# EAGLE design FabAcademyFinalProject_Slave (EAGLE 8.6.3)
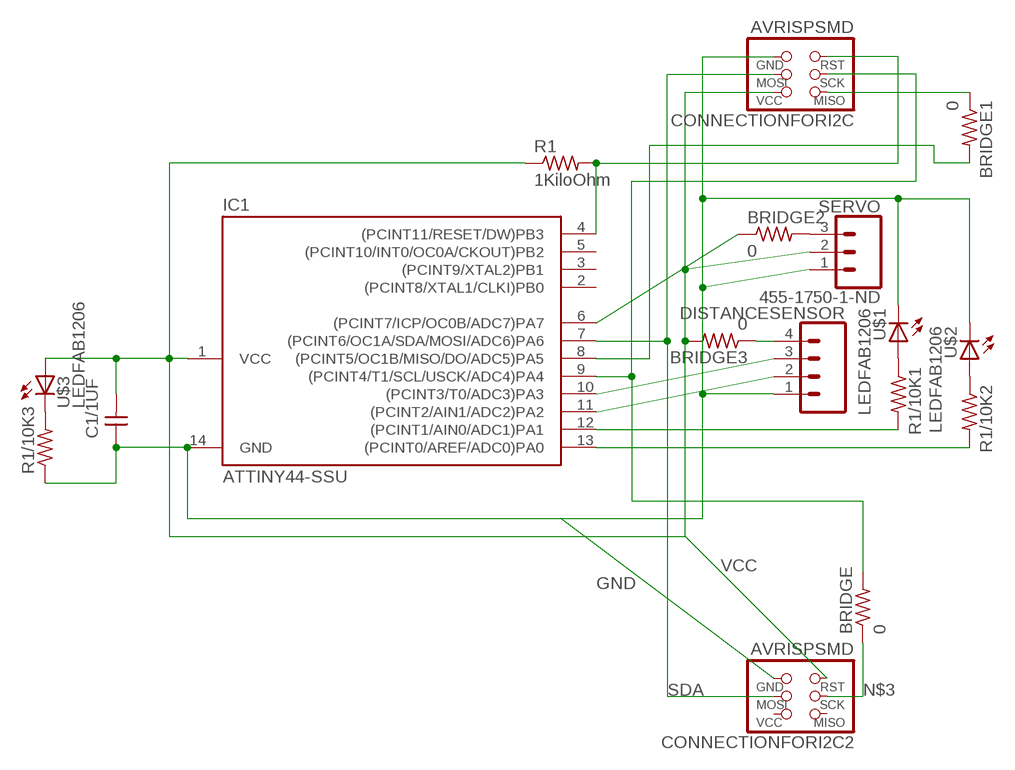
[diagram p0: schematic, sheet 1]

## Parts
BRIDGE  0  RES-US1206FAB  [R1206FAB]
BRIDGE1  0  RES-US1206FAB  [R1206FAB]
BRIDGE2  0  RES-US1206FAB  [R1206FAB]
BRIDGE3  0  RES-US1206FAB  [R1206FAB]
C1/1UF  CAP-UNPOLARIZEDFAB  [C1206FAB]
CONNECTIONFORI2C  AVRISPSMD  [2X03SMD]
CONNECTIONFORI2C2  AVRISPSMD  [2X03SMD]
DISTANCESENSOR  CONN_04  [1X04]
IC1  ATTINY44-SSU  [SOIC14]
R1  1KiloOhm  RES-US1206FAB  [R1206FAB]
R1/10K1  RES-US1206FAB  [R1206FAB]
R1/10K2  RES-US1206FAB  [R1206FAB]
R1/10K3  RES-US1206FAB  [R1206FAB]
SERVO  455-1750-1-ND  CONN_03  [1X03]
U$1  LEDFAB1206  [LED1206FAB]
U$2  LEDFAB1206  [LED1206FAB]
U$3  LEDFAB1206  [LED1206FAB]

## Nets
GND: C1/1UF.1 CONNECTIONFORI2C2.6(GND) CONNECTIONFORI2C.6(GND) DISTANCESENSOR.1 IC1.14(GND) R1/10K3.1 SERVO.1 U$1.2(C) U$2.2(C)
N$1: R1/10K2.1 U$2.1(A)
N$2: R1/10K3.2 U$3.2(C)
N$3: BRIDGE.1 CONNECTIONFORI2C2.3(SCK)
N$4: DISTANCESENSOR.3 IC1.10((PCINT3/T0/ADC3)PA3)
N$5: BRIDGE2.1 IC1.6((PCINT7/ICP/OC0B/ADC7)PA7)
N$6: BRIDGE1.2 IC1.8((PCINT5/OC1B/MISO/DO/ADC5)PA5)
N$7: CONNECTIONFORI2C.5(RST) IC1.4((PCINT11/RESET/DW)PB3) R1.2
N$8: IC1.13((PCINT0/AREF/ADC0)PA0) R1/10K2.2
N$9: IC1.12((PCINT1/AIN0/ADC1)PA1) R1/10K1.2
N$10: DISTANCESENSOR.2 IC1.11((PCINT2/AIN1/ADC2)PA2)
N$11: BRIDGE2.2 SERVO.3
N$12: R1/10K1.1 U$1.1(A)
N$13: BRIDGE3.1 DISTANCESENSOR.4
N$14: BRIDGE1.1 CONNECTIONFORI2C.1(MISO)
SCL: BRIDGE.2 CONNECTIONFORI2C.3(SCK) IC1.9((PCINT4/T1/SCL/USCK/ADC4)PA4)
SDA: CONNECTIONFORI2C2.4(MOSI) CONNECTIONFORI2C.4(MOSI) IC1.7((PCINT6/OC1A/SDA/MOSI/ADC6)PA6)
VCC: BRIDGE3.2 C1/1UF.2 CONNECTIONFORI2C2.5(RST) CONNECTIONFORI2C.2(VCC) IC1.1(VCC) R1.1 SERVO.2 U$3.1(A)
Unconnected: CONNECTIONFORI2C2.1(MISO) CONNECTIONFORI2C2.2(VCC) IC1.2((PCINT8/XTAL1/CLKI)PB0) IC1.3((PCINT9/XTAL2)PB1) IC1.5((PCINT10/INT0/OC0A/CKOUT)PB2)

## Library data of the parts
BRIDGE BRIDGE1-BRIDGE3 R1 R1/10K1-R1/10K3 = fab:RES-US: Resistor (US Symbol)
C1/1UF = fab:CAP-UNPOLARIZED
CONNECTIONFORI2C CONNECTIONFORI2C2 = fab:AVRISP
DISTANCESENSOR = SparkFun-Connectors:CONN_04: Multi connection point. Often used as Generic Header-pin footprint for 0.1 inch spaced/style header connections On any of the 0.1 inch spaced packages, you can populate with these: Break Away Headers - Straight (PRT-00116) Break Away Male Headers - Right Angle (PRT-00553) Female Headers (PRT-00115)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; PROD_ID: CONN-09696
IC1 = fab:ATTINY44
SERVO = SparkFun-Connectors:CONN_03: Multi connection point. Often used as Generic Header-pin footprint for 0.1 inch spaced/style header connections On any of the 0.1 inch spaced packages, you can populate with these: Break Away Headers - Straight (PRT-00116) Break Away Male Headers - Right Angle (PRT-00553) Female Headers (PRT-00115)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; PROD_ID: XXX-00000
U$1-U$3 = fab:LED: LED

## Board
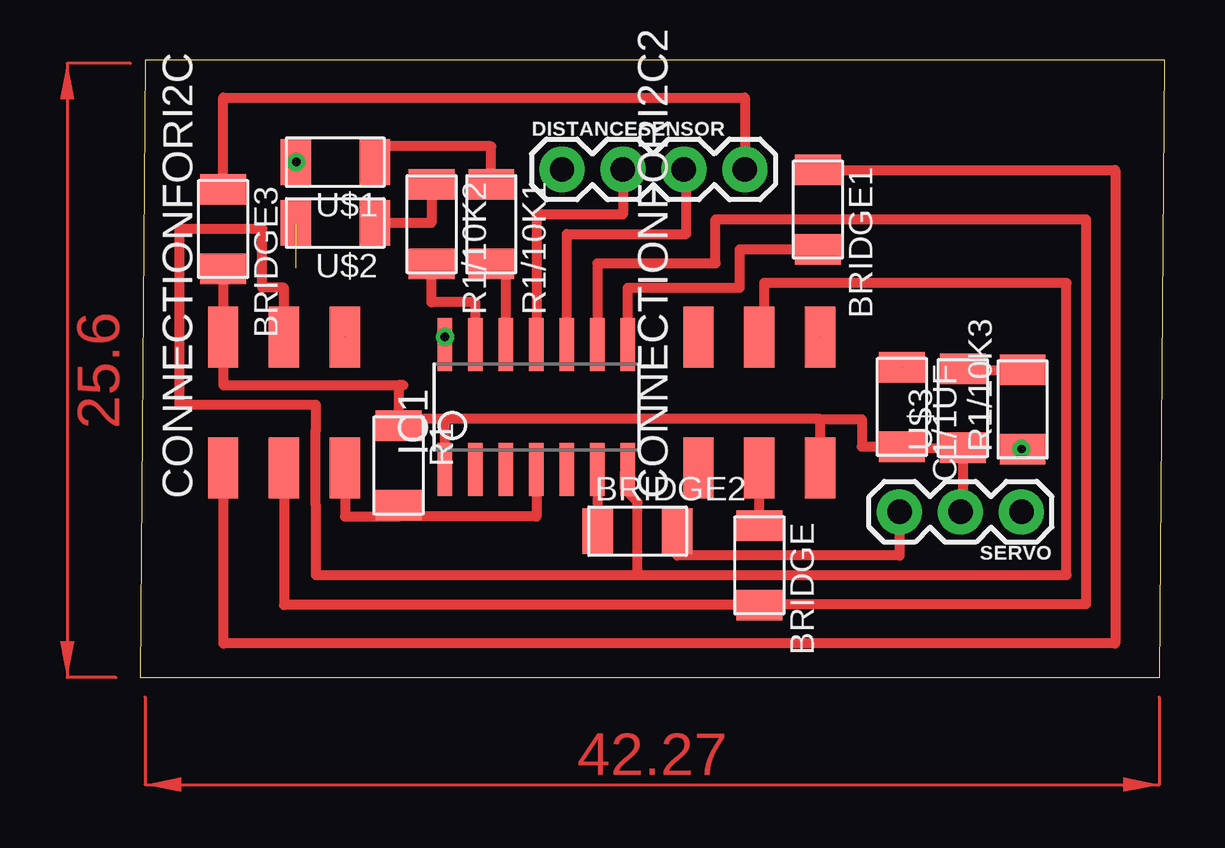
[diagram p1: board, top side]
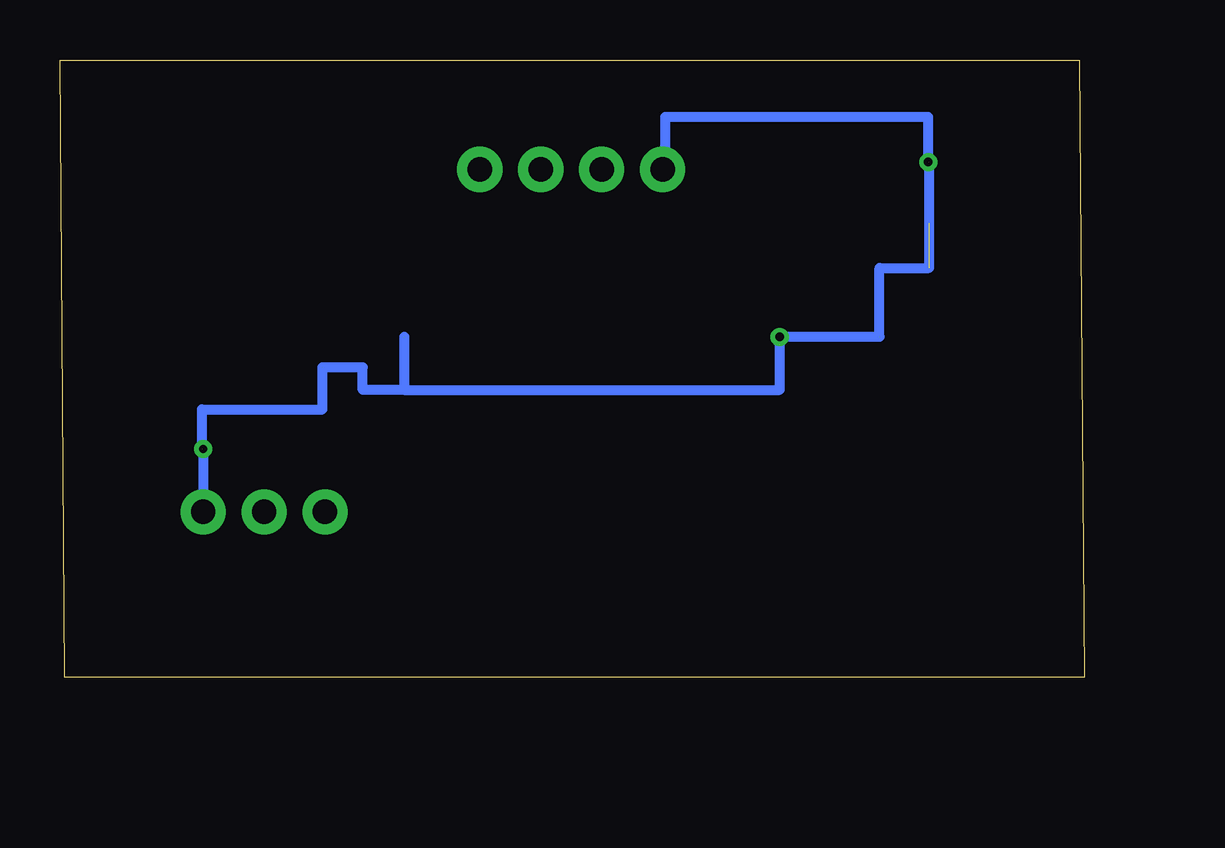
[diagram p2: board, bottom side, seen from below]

Size 42.7 x 25.75 mm. Coordinates in mm from the lower left corner, seen from the top.
Outline: 0,0 42.49,0 42.7,25.75 0.2,25.75 0,0
Copper layers (1*16): Top 0.035mm / dielectric 1.5mm / Bottom 0.035mm
Design rules "default *": minimum track width 6mil, minimum drill 0.35mm, track to track 16mil, track to pad 16mil, pad to pad 16mil, via to via 16mil, smd to smd 16mil, copper to edge 40mil, drill to drill 6mil, minimum pad ring 10mil, minimum via ring 8mil, stop-mask expansion 4mil, vias tented up to drill 0mil, thermal gap 10mil

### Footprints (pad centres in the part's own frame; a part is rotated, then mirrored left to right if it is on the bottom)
R1206FAB = smd 1.27 x 1.905: 1 -1.651,0; 2 1.651,0
C1206FAB = smd 1.27 x 1.905: 1 -1.651,0; 2 1.651,0
2X03SMD = smd 2.54 x 1.27: 1 -2.54,2.54; 2 2.92,2.54; 3 -2.54,0; 4 2.92,0; 5 -2.54,-2.54; 6 2.92,-2.54
1X04 = drill 1.016 pad 1.88: 1 0,0; 2 2.54,0; 3 5.08,0; 4 7.62,0
SOIC14 = smd 0.61 x 2.21: 1 -3.81,-2.603; 2 -2.54,-2.603; 3 -1.27,-2.603; 4 0,-2.603; 5 1.27,-2.603; 6 2.54,-2.603; 7 3.81,-2.603; 8 3.81,2.603; 9 2.54,2.603; 10 1.27,2.603; 11 0,2.603; 12 -1.27,2.603; 13 -2.54,2.603; 14 -3.81,2.603
1X03 = drill 1.016 pad 1.88: 1 0,0; 2 2.54,0; 3 5.08,0
LED1206FAB = smd 1.27 x 1.905: 1 -1.651,0; 2 1.651,0

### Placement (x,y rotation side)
BRIDGE  25.81,4.67 270 top
BRIDGE1  28.24,19.51 270 top
BRIDGE2  20.73,6.1 0 top
BRIDGE3  3.45,18.69 270 top
C1/1UF  31.75,11.28 270 top
CONNECTIONFORI2C  5.99,11.28 90 top
CONNECTIONFORI2C2  25.81,11.28 90 top
DISTANCESENSOR  17.58,21.18 0 top
IC1  16.51,11.28 0 top
R1  10.77,8.84 270 top
R1/10K1  14.63,18.9 270 top
R1/10K2  12.14,18.9 270 top
R1/10K3  36.78,11.18 90 top
SERVO  36.73,6.91 180 top
U$1  8.13,21.49 180 top
U$2  8.13,18.95 180 top
U$3  34.29,11.23 90 top

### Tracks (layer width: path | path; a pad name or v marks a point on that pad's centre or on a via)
GND  (via drill 0.35)  (7 unrouted)
  Top 0.406: v12.7,14.2 IC1.14 | R1/10K3.1 v36.73,9.52 | U$1.2 v6.5,21.49 | v17.48,21.18 DISTANCESENSOR.1
  Bottom 0.406: CONNECTIONFORI2C2.6 28.35,11.99 | 28.35,11.99 12.7,11.99 IC1.14 | 28.35,11.99 30.07,11.99 30.07,12.93 C1/1UF.1 31.75,11.18 36.78,11.18 R1/10K3.1 | U$1.2 6.48,17.07 8.53,17.07 CONNECTIONFORI2C.6 v12.7,14.2 | v36.73,9.52 SERVO.1 | v6.5,21.49 6.5,23.37 17.48,23.37 v17.48,21.18
N$1
  Top 0.406: R1/10K2.1 12.14,18.95 U$2.1
N$2
  Top 0.406: U$3.2 34.29,12.83 R1/10K3.2
N$3
  Top 0.406: BRIDGE.1 CONNECTIONFORI2C2.3
N$4
  Top 0.406: IC1.10 17.78,18.49 22.76,18.49 22.76,21.18 DISTANCESENSOR.3
N$5
  Top 0.406: IC1.6 19.05,6.1 BRIDGE2.1
N$6
  Top 0.406: IC1.8 20.32,16.26 24.99,16.26 24.99,17.86 BRIDGE1.2
N$7
  Top 0.406: IC1.4 16.51,6.71 10.77,6.71 | 10.77,6.71 R1.2 | CONNECTIONFORI2C.5 8.53,6.71 10.77,6.71
N$8
  Top 0.406: IC1.13 13.97,15.65 12.14,15.65 R1/10K2.2
N$9
  Top 0.406: IC1.12 15.24,17.27 14.63,17.27 R1/10K1.2
N$10
  Top 0.406: DISTANCESENSOR.2 20.12,19.3 16.51,19.3 IC1.11
N$11
  Top 0.406: BRIDGE2.2 22.38,5.08 31.65,5.08 SERVO.3
N$12
  Top 0.406: R1/10K1.1 14.63,22.15 9.78,22.15 U$1.1
N$13
  Top 0.406: BRIDGE3.1 3.45,24.18 25.2,24.18 DISTANCESENSOR.4
N$14
  Top 0.406: CONNECTIONFORI2C.1 3.45,1.42 40.64,1.42 40.64,21.16 BRIDGE1.1
SCL
  Top 0.406: CONNECTIONFORI2C.3 5.99,3.02 BRIDGE.2 25.81,3.05 39.42,3.05 39.42,19.1 23.98,19.1 23.98,17.27 23.77,17.27 19.05,17.27 IC1.9
SDA
  Top 0.406: CONNECTIONFORI2C.4 5.99,16.26 5.08,16.26 5.08,18.69 1.63,18.69 1.63,11.38 7.32,11.38 7.32,10.29 7.29,10.26 7.29,7.21 7.32,7.19 7.32,4.27 20.73,4.27 | CONNECTIONFORI2C2.4 26.01,14.2 26.01,16.46 38.61,16.46 38.61,4.27 20.73,4.27 | 20.73,4.27 20.73,7.32 20.21,7.83 20.21,8.57 IC1.7
VCC
  Top 0.406: CONNECTIONFORI2C2.5 28.35,10.77 | 28.35,10.77 12.7,10.77 | 28.35,10.77 30.07,10.77 30.07,9.63 C1/1UF.2 31.75,9.58 U$3.1 34.29,6.91 SERVO.2 | IC1.1 12.7,10.77 | 12.7,10.77 10.77,10.77 | 10.77,10.77 R1.1 | 10.97,12.19 10.77,12.19 | 10.77,12.19 10.77,10.77 | 10.77,12.19 3.45,12.19 CONNECTIONFORI2C.2 BRIDGE3.2
(copper drawn outside any net)
  shapes: Top area x2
